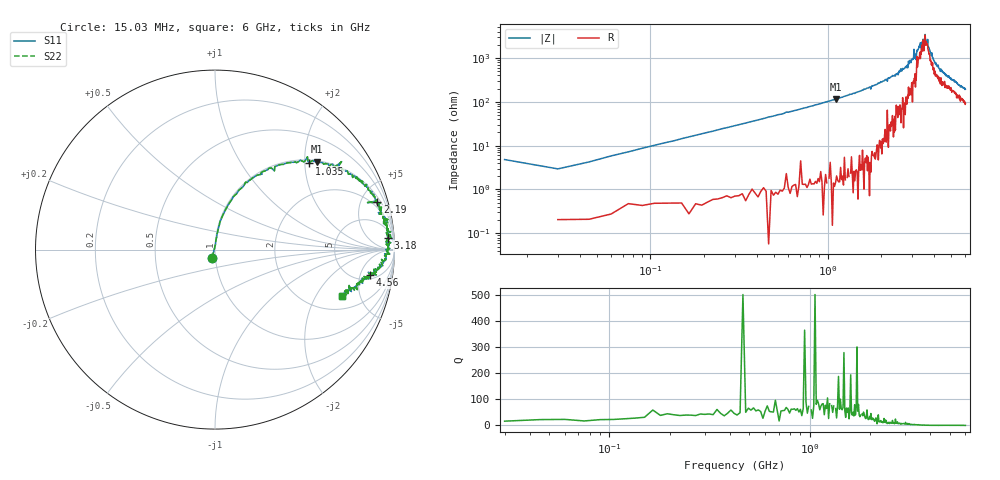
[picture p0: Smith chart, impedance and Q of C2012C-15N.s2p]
!	Network	Analyzer	HP8753E.07.74:	Oct	30	2002	Serial	No.	JP38451487
!	Hewlett-Packard
!	7	Sep	2009	10:45:36
!	Frequency	S11	S21	S12	S22
#	HZ	S	RI	R	50
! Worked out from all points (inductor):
!   400 points, 15.03 MHz to 6 GHz, reference 50 ohm
!   read as one part in series: L = 15.3 nH near 45.03 MHz
!   highest Q = 79.9 at 1.11 GHz (marker M1), where L = 16.5 nH
!   self-resonance near 3.51 GHz
!   S11 on the Smith chart (normalised r, x): 15.03 MHz: 0.96, -0.09; 1.035 GHz: 1.08, +2.11; 2.19 GHz: 1.41, +6.71; 3.18 GHz: 12, +23; 4.56 GHz: 6.04, -7.35; 6 GHz: 2.82, -3.40
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1.502992e7  -0.0158 -0.0457  1.02 0.0457  1.02 0.0457  -0.0158 -0.0457
3.002985e7  0.00282 0.0293  0.997 -0.0293  0.997 -0.0293  0.00282 0.0293
1.200294e8  0.0177 0.113  0.982 -0.113  0.982 -0.113  0.0177 0.113
3.150284e8  0.0889 0.273  0.911 -0.273  0.911 -0.273  0.0889 0.273
1.020025e9  0.518 0.491  0.482 -0.491  0.482 -0.491  0.518 0.491
1.035025e9  0.526 0.48  0.474 -0.48  0.474 -0.48  0.526 0.48
1.110024e9  0.569 0.489  0.431 -0.489  0.431 -0.489  0.569 0.489
2.01002e9  0.88 0.304  0.12 -0.304  0.12 -0.304  0.88 0.304
2.190019e9  0.905 0.264  0.0955 -0.264  0.0955 -0.264  0.905 0.264
3.015015e9  0.979 0.0998  0.0207 -0.0998  0.0207 -0.0998  0.979 0.0998
3.075015e9  0.986 0.0609  0.0144 -0.0609  0.0144 -0.0609  0.986 0.0609
3.105014e9  0.961 0.0894  0.0388 -0.0894  0.0388 -0.0894  0.961 0.0894
3.180014e9  0.963 0.0653  0.0369 -0.0653  0.0369 -0.0653  0.963 0.0653
3.525012e9  0.956 -0.0116  0.0438 0.0116  0.0438 0.0116  0.956 -0.0116
3.555012e9  0.973 0.00699  0.0274 -0.00699  0.0274 -0.00699  0.973 0.00699
3.585012e9  0.951 0.00137  0.0486 -0.00137  0.0486 -0.00137  0.951 0.00137
3.675012e9  0.973 -0.0245  0.0273 0.0245  0.0273 0.0245  0.973 -0.0245
3.705011e9  0.945 -0.0229  0.0546 0.0229  0.0546 0.0229  0.945 -0.0229
4.00501e9  0.934 -0.0901  0.0656 0.0901  0.0656 0.0901  0.934 -0.0901
4.560007e9  0.864 -0.142  0.136 0.142  0.136 0.142  0.864 -0.142
5.010005e9  0.817 -0.172  0.183 0.172  0.183 0.172  0.817 -0.172
6e9  0.708 -0.26  0.292 0.26  0.292 0.26  0.708 -0.26
